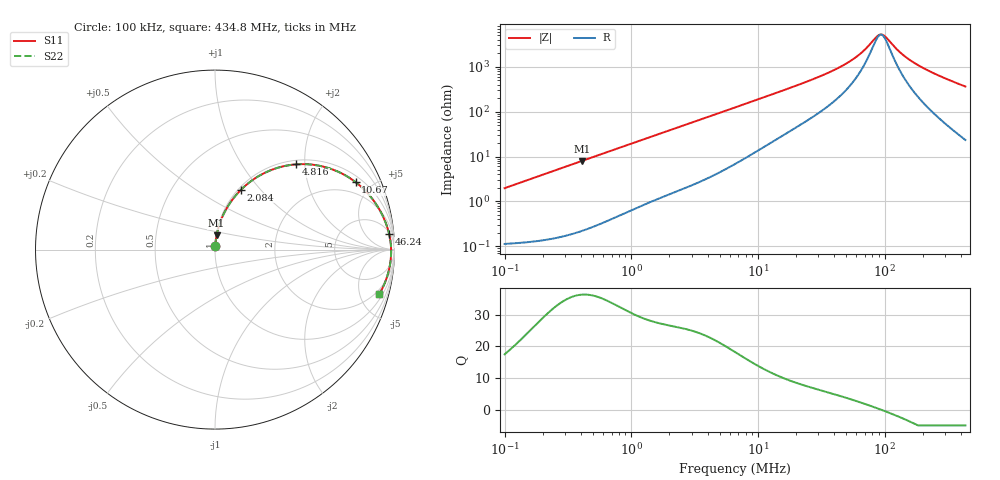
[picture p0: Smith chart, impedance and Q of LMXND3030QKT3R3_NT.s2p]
! LMXND3030QKT3R3_NT  S-PARAMETER MODEL  ( Standard Model )
! Model Generated by TAIYO YUDEN Corporation (https://www.yuden.co.jp/en/)
! Version 1.0
! TAIYO YUDEN Control No. 20250925
! Copyright(c) 2025 TAIYO YUDEN CO.,LTD. All Rights Reserved.
! Product Description (link to TY-COMPAS)
! https://ds.yuden.co.jp/TYCOMPAS/or/detail?pn=LMXND3030QKT3R3MNT&u=M
! Products Name : Inductors
! Characteristics :
!  Inductance : 3.3 [uH] , SRF(min) : 49 [MHz] , DC Resistance(max) : 0.094 [Ohm]
!  Rated Current : Saturation  1210 [mA] , Temp Rise  1900 [mA] (40 [degC])
!  Case Size : 3.0 x 3.0 / 0.118 x 0.118 [mm/inch] , Thickness : 1.5 / 0.059 [mm/inch]
!  (Conditions: Temperature = 25 [degC] , DC Bias Current = 0 [A])
! External Node Assignments :
!  1  o---GGG---o  2
! GND o---------o GND
! Frequency Range : 0.1MHz  -  434.768421MHz  [ 402 STEP ]
# MHz S RI R 50
! Freq[MHz].  S11 Real  S11 Imag  S21 Real  S21 Imag  S12 Real  S12 Imag  S22 Real  S22 Imag
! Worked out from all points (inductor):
!   401 points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, 100 kHz to 434.8 MHz, reference 50 ohm
!   read as one part in series: L = 3.13 uH near 104.3 kHz
!   highest Q = 36.3 at 406.8 kHz (marker M1), where L = 3.12 uH
!   self-resonance near 93.52 MHz
!   S11 on the Smith chart (normalised r, x): 100 kHz: 1.00, +0.04; 2.084 MHz: 1.03, +0.79; 4.816 MHz: 1.08, +1.81; 10.67 MHz: 1.30, +4.00; 46.24 MHz: 6, +20; 434.8 MHz: 1.47, -7.25
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0.1  0.00151 0.0197  0.9985 -0.0197  0.9985 -0.0197  0.00151 0.0197
0.406826  0.00845 0.0788  0.9916 -0.0788  0.9916 -0.0788  0.00845 0.0788
0.846751  0.031 0.1585  0.969 -0.1585  0.969 -0.1585  0.031 0.1585
1.65507  0.0998 0.282  0.9002 -0.282  0.9002 -0.282  0.0998 0.282
2.08386  0.1456 0.3343  0.8544 -0.3343  0.8544 -0.3343  0.1456 0.3343
3.102314  0.265 0.4216  0.735 -0.4216  0.735 -0.4216  0.265 0.4216
4.816087  0.454 0.4751  0.546 -0.4751  0.546 -0.4751  0.454 0.4751
6.733248  0.61 0.4607  0.39 -0.4607  0.39 -0.4607  0.61 0.4607
10.67404  0.7835 0.3758  0.2165 -0.3758  0.2165 -0.3758  0.7835 0.3758
16.22713  0.8804 0.2775  0.1196 -0.2775  0.1196 -0.2775  0.8804 0.2775
26.82484  0.9408 0.1742  0.0592 -0.1742  0.0592 -0.1742  0.9408 0.1742
46.24065  0.97 0.088  0.03 -0.088  0.03 -0.088  0.97 0.088
63.30801  0.9776 0.0469  0.0224 -0.0469  0.0224 -0.0469  0.9776 0.0469
71.78481  0.9794 0.0315  0.0206 -0.0315  0.0206 -0.0315  0.9794 0.0315
84.8785  0.9809 0.0115  0.0191 -0.0115  0.0191 -0.0115  0.9809 0.0115
90.38256  0.9812 0.00405  0.0188 -0.00405  0.0188 -0.00405  0.9812 0.00405
98.28046  0.9814 -0.0059  0.0186 0.0059  0.0186 0.0059  0.9814 -0.0059
109.1303  0.9813 -0.0184  0.0187 0.0184  0.0187 0.0184  0.9813 -0.0184
137.4034  0.9798 -0.0469  0.0202 0.0469  0.0202 0.0469  0.9798 -0.0469
180.4018  0.9752 -0.0836  0.0248 0.0836  0.0248 0.0836  0.9752 -0.0836
268.5704  0.9599 -0.1474  0.0401 0.1474  0.0401 0.1474  0.9599 -0.1474
434.7684  0.9159 -0.2472  0.0841 0.2472  0.0841 0.2472  0.9159 -0.2472
